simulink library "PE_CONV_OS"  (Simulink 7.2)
settings: Solver=ode45  SolverMode=SingleTasking  StartTime=0.0  StopTime=10.0  RelTol=1e-3
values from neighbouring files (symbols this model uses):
  C = 10e-3*1    (= 0.01)    [INIT_B6_2L_3Ph_IGBT_OS.m]    (also in INIT_B6_3L_3Ph_IGBT_OS.m; INIT_MMC_100L.m = 0.005; INIT_MMC_200L.m = 0.005; INIT_MMC_20L.m)
  FS = 900    [INIT_B6_2L_3Ph_IGBT_OS.m]    (also in INIT_B6_3L_3Ph_IGBT_OS.m; INIT_PWM_2L.m = 1000; INIT_PWM_3L.m = 1000; INIT_PWM_Con.m = 1000)
  LN = 2e-3    (= 0.002)    [INIT_PWM_2L.m]    (also in INIT_PWM_3L.m; INIT_PWM_Con.m; INIT_MMC_100L.m = 0.025; INIT_MMC_200L.m = 0.025)
  LS = 1e-3    (= 0.001)    [INIT_B6_2L_3Ph_IGBT_OS.m]    (also in INIT_B6_3L_3Ph_IGBT_OS.m; INIT_MMC_100L.m = 0.025; INIT_MMC_200L.m = 0.025; INIT_MMC_20L.m = 0.0025)
  LT = LN    (= 0.025)    [INIT_MMC_100L.m]    (also in INIT_MMC_200L.m; INIT_MMC_20L.m = 0.002; INIT_MMC_400L.m)
  Nc = 100    [INIT_MMC_100L.m]    (also in INIT_MMC_200L.m = 200; INIT_MMC_20L.m = 20; INIT_MMC_400L.m = 400)
  NT = sqrt(3)*340/400    [INIT_MMC_100L.m]    (also in INIT_MMC_200L.m; INIT_MMC_20L.m = sqrt(3); INIT_MMC_400L.m)
  Rg = 1e-3    (= 0.001)    [INIT_MMC_100L.m]    (also in INIT_MMC_200L.m; INIT_MMC_20L.m; INIT_MMC_400L.m)
  RN = 0.1    [INIT_PWM_2L.m]    (also in INIT_PWM_3L.m; INIT_PWM_Con.m; INIT_MMC_100L.m; INIT_MMC_200L.m)
  RT = RN    (= 0.1)    [INIT_MMC_100L.m]    (also in INIT_MMC_200L.m; INIT_MMC_20L.m; INIT_MMC_400L.m)
  UC0 = 600    [INIT_B6_2L_3Ph_IGBT_OS.m]    (also in INIT_B6_3L_3Ph_IGBT_OS.m = 500; INIT_MMC_100L.m = 6800; INIT_MMC_200L.m = 3400; INIT_MMC_20L.m = 5000)
undefined symbols (not defined in the file or in its folder): A, DT, FT, L, O1, O2, PHT, T, Td
libraries: simulink_extras x2
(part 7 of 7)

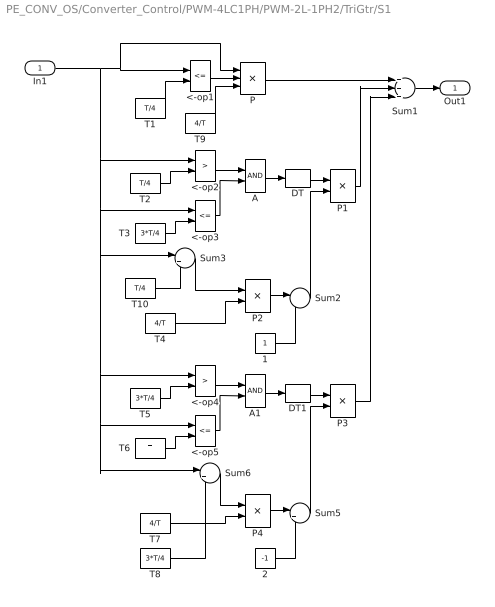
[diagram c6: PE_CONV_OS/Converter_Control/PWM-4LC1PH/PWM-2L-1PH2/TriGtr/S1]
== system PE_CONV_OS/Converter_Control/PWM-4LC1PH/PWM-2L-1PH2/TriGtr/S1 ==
  In1 : Inport  OutDataType=sfix(16)  OutScaling=2^0
  1 : Constant  OutDataType=sfix(16)  OutScaling=2^0
  2 : Constant  Value=-1  OutDataType=sfix(16)  OutScaling=2^0
  <-op1 : RelationalOperator  Operator=<=
  <-op2 : RelationalOperator  Operator=>
  <-op3 : RelationalOperator  Operator=<=
  <-op4 : RelationalOperator  Operator=>
  <-op5 : RelationalOperator  Operator=<=
  A : Logic  AllPortsSameDT=off
  A1 : Logic  AllPortsSameDT=off
  DT : DataTypeConversion
  DT1 : DataTypeConversion
  P : Product  Inputs=3  OutDataType=sfix(16)  OutScaling=2^0
  P{1..4} (4 alike) : Product  OutDataType=sfix(16)  OutScaling=2^0
  Sum1 : Sum  Inputs=+++  OutDataType=sfix(16)  OutScaling=2^0
  Sum2 : Sum  Inputs=|-+  OutDataType=sfix(16)  OutScaling=2^0
  Sum3 : Sum  Inputs=|+-  OutDataType=sfix(16)  OutScaling=2^0
  Sum5 : Sum  Inputs=|++  OutDataType=sfix(16)  OutScaling=2^0
  Sum6 : Sum  Inputs=|+-  OutDataType=sfix(16)  OutScaling=2^0
  T1 : Constant  Value=T/4  OutDataType=sfix(16)  OutScaling=2^0
  T10 : Constant  Value=T/4  OutDataType=sfix(16)  OutScaling=2^0
  T2 : Constant  Value=T/4  OutDataType=sfix(16)  OutScaling=2^0
  T3 : Constant  Value=3*T/4  OutDataType=sfix(16)  OutScaling=2^0
  T4 : Constant  Value=4/T  OutDataType=sfix(16)  OutScaling=2^0
  T5 : Constant  Value=3*T/4  OutDataType=sfix(16)  OutScaling=2^0
  T6 : Constant  Value=T  OutDataType=sfix(16)  OutScaling=2^0
  T7 : Constant  Value=4/T  OutDataType=sfix(16)  OutScaling=2^0
  T8 : Constant  Value=3*T/4  OutDataType=sfix(16)  OutScaling=2^0
  T9 : Constant  Value=4/T  OutDataType=sfix(16)  OutScaling=2^0
  Out1 : Outport
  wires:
  T10/1 -> Sum3/2
  T9/1 -> P/3
  DT1/1 -> P3/1
  DT/1 -> P1/1
  T1/1 -> <-op1/2
  <-op1/1 -> P/2
  P/1 -> Sum1/1
  T2/1 -> <-op2/2
  <-op2/1 -> A/1
  T3/1 -> <-op3/2
  <-op3/1 -> A/2
  A/1 -> DT/1
  T4/1 -> P2/2
  Sum3/1 -> P2/1
  In1/1 -> <-op2/1, <-op3/1, Sum3/1, <-op4/1, <-op5/1, Sum6/1, <-op1/1, P/1
  P1/1 -> Sum1/2
  P2/1 -> Sum2/1
  1/1 -> Sum2/2
  Sum2/1 -> P1/2
  T5/1 -> <-op4/2
  <-op4/1 -> A1/1
  T6/1 -> <-op5/2
  <-op5/1 -> A1/2
  A1/1 -> DT1/1
  T7/1 -> P4/2
  Sum6/1 -> P4/1
  P4/1 -> Sum5/1
  2/1 -> Sum5/2
  Sum5/1 -> P3/2
  T8/1 -> Sum6/2
  P3/1 -> Sum1/3
  Sum1/1 -> Out1/1

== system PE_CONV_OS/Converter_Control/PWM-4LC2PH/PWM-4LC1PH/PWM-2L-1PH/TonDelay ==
  s1 : Inport  Orientation=down  OutDataType=sfix(16)  OutScaling=2^0
  Int : Integrator  ExternalReset=falling
  Rel1 : Relay  OnSwitchValue=DT  OutDataType=sfix(16)  OutScaling=2^0
  s1d : Outport  InitialOutput=0
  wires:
  Rel1/1 -> s1d/1
  s1/1 -> Int/1, Int/2
  Int/1 -> Rel1/1

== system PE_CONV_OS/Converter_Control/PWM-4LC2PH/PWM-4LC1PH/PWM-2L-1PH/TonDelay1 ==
  s1 : Inport  Orientation=down  OutDataType=sfix(16)  OutScaling=2^0
  Int : Integrator  ExternalReset=falling
  Rel1 : Relay  OnSwitchValue=DT  OutDataType=sfix(16)  OutScaling=2^0
  s1d : Outport  InitialOutput=0
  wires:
  Rel1/1 -> s1d/1
  s1/1 -> Int/1, Int/2
  Int/1 -> Rel1/1

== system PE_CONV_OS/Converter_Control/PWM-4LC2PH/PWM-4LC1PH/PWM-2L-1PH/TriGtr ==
  Clock : Clock
  S1 : Subsystem
  Sum : Sum  OutDataType=sfix(16)  OutScaling=2^0
  T : Constant  Value=T  OutDataType=sfix(16)  OutScaling=2^0
  Td : Constant  Value=Td  OutDataType=sfix(16)  OutScaling=2^0
  mod : Math  Operator=mod
  O : Outport  InitialOutput=0
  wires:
  Td/1 -> Sum/2
  Sum/1 -> mod/1
  T/1 -> mod/2
  Clock/1 -> Sum/1
  S1/1(Out1) -> O/1
  mod/1 -> S1/1(In1)

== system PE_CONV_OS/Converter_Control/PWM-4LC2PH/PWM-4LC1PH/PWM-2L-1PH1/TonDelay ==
  s1 : Inport  Orientation=down  OutDataType=sfix(16)  OutScaling=2^0
  Int : Integrator  ExternalReset=falling
  Rel1 : Relay  OnSwitchValue=DT  OutDataType=sfix(16)  OutScaling=2^0
  s1d : Outport  InitialOutput=0
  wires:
  Int/1 -> Rel1/1
  s1/1 -> Int/2, Int/1
  Rel1/1 -> s1d/1

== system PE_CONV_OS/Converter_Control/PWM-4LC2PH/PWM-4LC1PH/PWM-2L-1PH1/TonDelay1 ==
  s1 : Inport  Orientation=down  OutDataType=sfix(16)  OutScaling=2^0
  Int : Integrator  ExternalReset=falling
  Rel1 : Relay  OnSwitchValue=DT  OutDataType=sfix(16)  OutScaling=2^0
  s1d : Outport  InitialOutput=0
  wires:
  Int/1 -> Rel1/1
  s1/1 -> Int/2, Int/1
  Rel1/1 -> s1d/1

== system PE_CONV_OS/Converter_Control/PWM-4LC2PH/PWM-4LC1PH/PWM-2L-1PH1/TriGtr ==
  Clock : Clock
  S1 : Subsystem
  Sum : Sum  OutDataType=sfix(16)  OutScaling=2^0
  T : Constant  Value=T  OutDataType=sfix(16)  OutScaling=2^0
  Td : Constant  Value=Td  OutDataType=sfix(16)  OutScaling=2^0
  mod : Math  Operator=mod
  O : Outport  InitialOutput=0
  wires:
  mod/1 -> S1/1(In1)
  S1/1(Out1) -> O/1
  Clock/1 -> Sum/1
  T/1 -> mod/2
  Sum/1 -> mod/1
  Td/1 -> Sum/2

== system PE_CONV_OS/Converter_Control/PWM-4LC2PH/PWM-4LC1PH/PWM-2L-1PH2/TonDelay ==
  s1 : Inport  Orientation=down  OutDataType=sfix(16)  OutScaling=2^0
  Int : Integrator  ExternalReset=falling
  Rel1 : Relay  OnSwitchValue=DT  OutDataType=sfix(16)  OutScaling=2^0
  s1d : Outport  InitialOutput=0
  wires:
  Rel1/1 -> s1d/1
  s1/1 -> Int/1, Int/2
  Int/1 -> Rel1/1

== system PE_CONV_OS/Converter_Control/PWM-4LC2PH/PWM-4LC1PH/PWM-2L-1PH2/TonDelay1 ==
  s1 : Inport  Orientation=down  OutDataType=sfix(16)  OutScaling=2^0
  Int : Integrator  ExternalReset=falling
  Rel1 : Relay  OnSwitchValue=DT  OutDataType=sfix(16)  OutScaling=2^0
  s1d : Outport  InitialOutput=0
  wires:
  Rel1/1 -> s1d/1
  s1/1 -> Int/1, Int/2
  Int/1 -> Rel1/1

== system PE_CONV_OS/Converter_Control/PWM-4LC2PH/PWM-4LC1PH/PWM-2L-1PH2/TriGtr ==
  Clock : Clock
  S1 : Subsystem
  Sum : Sum  OutDataType=sfix(16)  OutScaling=2^0
  T : Constant  Value=T  OutDataType=sfix(16)  OutScaling=2^0
  Td : Constant  Value=Td  OutDataType=sfix(16)  OutScaling=2^0
  mod : Math  Operator=mod
  O : Outport  InitialOutput=0
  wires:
  Td/1 -> Sum/2
  Sum/1 -> mod/1
  T/1 -> mod/2
  Clock/1 -> Sum/1
  S1/1(Out1) -> O/1
  mod/1 -> S1/1(In1)

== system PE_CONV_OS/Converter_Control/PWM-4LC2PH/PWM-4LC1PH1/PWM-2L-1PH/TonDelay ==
  s1 : Inport  Orientation=down  OutDataType=sfix(16)  OutScaling=2^0
  Int : Integrator  ExternalReset=falling
  Rel1 : Relay  OnSwitchValue=DT  OutDataType=sfix(16)  OutScaling=2^0
  s1d : Outport  InitialOutput=0
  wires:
  Int/1 -> Rel1/1
  s1/1 -> Int/2, Int/1
  Rel1/1 -> s1d/1

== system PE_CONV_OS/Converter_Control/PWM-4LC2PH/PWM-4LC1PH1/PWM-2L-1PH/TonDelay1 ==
  s1 : Inport  Orientation=down  OutDataType=sfix(16)  OutScaling=2^0
  Int : Integrator  ExternalReset=falling
  Rel1 : Relay  OnSwitchValue=DT  OutDataType=sfix(16)  OutScaling=2^0
  s1d : Outport  InitialOutput=0
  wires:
  Int/1 -> Rel1/1
  s1/1 -> Int/2, Int/1
  Rel1/1 -> s1d/1

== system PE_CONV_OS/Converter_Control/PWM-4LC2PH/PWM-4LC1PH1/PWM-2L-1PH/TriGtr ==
  Clock : Clock
  S1 : Subsystem
  Sum : Sum  OutDataType=sfix(16)  OutScaling=2^0
  T : Constant  Value=T  OutDataType=sfix(16)  OutScaling=2^0
  Td : Constant  Value=Td  OutDataType=sfix(16)  OutScaling=2^0
  mod : Math  Operator=mod
  O : Outport  InitialOutput=0
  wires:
  mod/1 -> S1/1(In1)
  S1/1(Out1) -> O/1
  Clock/1 -> Sum/1
  T/1 -> mod/2
  Sum/1 -> mod/1
  Td/1 -> Sum/2

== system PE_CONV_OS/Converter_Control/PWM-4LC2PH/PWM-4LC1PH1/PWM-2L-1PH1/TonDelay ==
  s1 : Inport  Orientation=down  OutDataType=sfix(16)  OutScaling=2^0
  Int : Integrator  ExternalReset=falling
  Rel1 : Relay  OnSwitchValue=DT  OutDataType=sfix(16)  OutScaling=2^0
  s1d : Outport  InitialOutput=0
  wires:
  Rel1/1 -> s1d/1
  s1/1 -> Int/1, Int/2
  Int/1 -> Rel1/1

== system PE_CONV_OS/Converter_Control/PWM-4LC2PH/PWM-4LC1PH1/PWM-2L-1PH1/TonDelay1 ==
  s1 : Inport  Orientation=down  OutDataType=sfix(16)  OutScaling=2^0
  Int : Integrator  ExternalReset=falling
  Rel1 : Relay  OnSwitchValue=DT  OutDataType=sfix(16)  OutScaling=2^0
  s1d : Outport  InitialOutput=0
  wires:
  Rel1/1 -> s1d/1
  s1/1 -> Int/1, Int/2
  Int/1 -> Rel1/1

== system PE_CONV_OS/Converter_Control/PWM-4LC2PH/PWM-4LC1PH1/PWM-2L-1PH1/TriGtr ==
  Clock : Clock
  S1 : Subsystem
  Sum : Sum  OutDataType=sfix(16)  OutScaling=2^0
  T : Constant  Value=T  OutDataType=sfix(16)  OutScaling=2^0
  Td : Constant  Value=Td  OutDataType=sfix(16)  OutScaling=2^0
  mod : Math  Operator=mod
  O : Outport  InitialOutput=0
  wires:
  Td/1 -> Sum/2
  Sum/1 -> mod/1
  T/1 -> mod/2
  Clock/1 -> Sum/1
  S1/1(Out1) -> O/1
  mod/1 -> S1/1(In1)

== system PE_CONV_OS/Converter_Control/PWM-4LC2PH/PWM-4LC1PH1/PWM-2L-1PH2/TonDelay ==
  s1 : Inport  Orientation=down  OutDataType=sfix(16)  OutScaling=2^0
  Int : Integrator  ExternalReset=falling
  Rel1 : Relay  OnSwitchValue=DT  OutDataType=sfix(16)  OutScaling=2^0
  s1d : Outport  InitialOutput=0
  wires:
  Int/1 -> Rel1/1
  s1/1 -> Int/2, Int/1
  Rel1/1 -> s1d/1

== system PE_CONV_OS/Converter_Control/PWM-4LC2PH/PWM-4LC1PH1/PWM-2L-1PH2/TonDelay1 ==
  s1 : Inport  Orientation=down  OutDataType=sfix(16)  OutScaling=2^0
  Int : Integrator  ExternalReset=falling
  Rel1 : Relay  OnSwitchValue=DT  OutDataType=sfix(16)  OutScaling=2^0
  s1d : Outport  InitialOutput=0
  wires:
  Int/1 -> Rel1/1
  s1/1 -> Int/2, Int/1
  Rel1/1 -> s1d/1

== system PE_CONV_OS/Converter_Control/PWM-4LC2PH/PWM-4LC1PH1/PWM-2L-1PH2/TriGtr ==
  Clock : Clock
  S1 : Subsystem
  Sum : Sum  OutDataType=sfix(16)  OutScaling=2^0
  T : Constant  Value=T  OutDataType=sfix(16)  OutScaling=2^0
  Td : Constant  Value=Td  OutDataType=sfix(16)  OutScaling=2^0
  mod : Math  Operator=mod
  O : Outport  InitialOutput=0
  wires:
  mod/1 -> S1/1(In1)
  S1/1(Out1) -> O/1
  Clock/1 -> Sum/1
  T/1 -> mod/2
  Sum/1 -> mod/1
  Td/1 -> Sum/2

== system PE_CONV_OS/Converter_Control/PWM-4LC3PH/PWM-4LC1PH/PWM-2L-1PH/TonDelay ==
  s1 : Inport  Orientation=down  OutDataType=sfix(16)  OutScaling=2^0
  Int : Integrator  ExternalReset=falling
  Rel1 : Relay  OnSwitchValue=DT  OutDataType=sfix(16)  OutScaling=2^0
  s1d : Outport  InitialOutput=0
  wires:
  Rel1/1 -> s1d/1
  s1/1 -> Int/1, Int/2
  Int/1 -> Rel1/1

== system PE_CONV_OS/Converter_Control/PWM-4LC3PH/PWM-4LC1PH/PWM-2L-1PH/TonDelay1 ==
  s1 : Inport  Orientation=down  OutDataType=sfix(16)  OutScaling=2^0
  Int : Integrator  ExternalReset=falling
  Rel1 : Relay  OnSwitchValue=DT  OutDataType=sfix(16)  OutScaling=2^0
  s1d : Outport  InitialOutput=0
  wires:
  Rel1/1 -> s1d/1
  s1/1 -> Int/1, Int/2
  Int/1 -> Rel1/1

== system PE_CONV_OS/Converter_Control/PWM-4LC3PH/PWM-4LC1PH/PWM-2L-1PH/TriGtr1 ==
  Clock : Clock
  S1 : Subsystem
  Sum : Sum  OutDataType=sfix(16)  OutScaling=2^0
  T : Constant  Value=T  OutDataType=sfix(16)  OutScaling=2^0
  Td : Constant  Value=Td  OutDataType=sfix(16)  OutScaling=2^0
  mod : Math  Operator=mod
  O : Outport  InitialOutput=0
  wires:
  Td/1 -> Sum/2
  Sum/1 -> mod/1
  T/1 -> mod/2
  Clock/1 -> Sum/1
  S1/1(O1) -> O/1
  mod/1 -> S1/1(I1)

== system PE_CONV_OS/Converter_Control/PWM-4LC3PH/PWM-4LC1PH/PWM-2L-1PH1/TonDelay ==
  s1 : Inport  Orientation=down  OutDataType=sfix(16)  OutScaling=2^0
  Int : Integrator  ExternalReset=falling
  Rel1 : Relay  OnSwitchValue=DT  OutDataType=sfix(16)  OutScaling=2^0
  s1d : Outport  InitialOutput=0
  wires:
  Int/1 -> Rel1/1
  s1/1 -> Int/2, Int/1
  Rel1/1 -> s1d/1

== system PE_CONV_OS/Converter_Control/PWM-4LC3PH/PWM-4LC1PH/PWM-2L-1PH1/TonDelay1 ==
  s1 : Inport  Orientation=down  OutDataType=sfix(16)  OutScaling=2^0
  Int : Integrator  ExternalReset=falling
  Rel1 : Relay  OnSwitchValue=DT  OutDataType=sfix(16)  OutScaling=2^0
  s1d : Outport  InitialOutput=0
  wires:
  Int/1 -> Rel1/1
  s1/1 -> Int/2, Int/1
  Rel1/1 -> s1d/1

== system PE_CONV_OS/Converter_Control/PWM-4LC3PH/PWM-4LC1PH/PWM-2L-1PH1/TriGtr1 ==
  Clock : Clock
  S1 : Subsystem
  Sum : Sum  OutDataType=sfix(16)  OutScaling=2^0
  T : Constant  Value=T  OutDataType=sfix(16)  OutScaling=2^0
  Td : Constant  Value=Td  OutDataType=sfix(16)  OutScaling=2^0
  mod : Math  Operator=mod
  O : Outport  InitialOutput=0
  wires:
  mod/1 -> S1/1(I1)
  S1/1(O1) -> O/1
  Clock/1 -> Sum/1
  T/1 -> mod/2
  Sum/1 -> mod/1
  Td/1 -> Sum/2

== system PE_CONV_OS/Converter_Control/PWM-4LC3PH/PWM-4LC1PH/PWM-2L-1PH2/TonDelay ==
  s1 : Inport  Orientation=down  OutDataType=sfix(16)  OutScaling=2^0
  Int : Integrator  ExternalReset=falling
  Rel1 : Relay  OnSwitchValue=DT  OutDataType=sfix(16)  OutScaling=2^0
  s1d : Outport  InitialOutput=0
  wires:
  Rel1/1 -> s1d/1
  s1/1 -> Int/1, Int/2
  Int/1 -> Rel1/1

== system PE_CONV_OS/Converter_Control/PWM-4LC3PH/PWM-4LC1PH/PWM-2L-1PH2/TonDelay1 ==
  s1 : Inport  Orientation=down  OutDataType=sfix(16)  OutScaling=2^0
  Int : Integrator  ExternalReset=falling
  Rel1 : Relay  OnSwitchValue=DT  OutDataType=sfix(16)  OutScaling=2^0
  s1d : Outport  InitialOutput=0
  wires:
  Rel1/1 -> s1d/1
  s1/1 -> Int/1, Int/2
  Int/1 -> Rel1/1

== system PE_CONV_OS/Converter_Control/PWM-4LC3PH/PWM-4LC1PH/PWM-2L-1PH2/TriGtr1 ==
  Clock : Clock
  S1 : Subsystem
  Sum : Sum  OutDataType=sfix(16)  OutScaling=2^0
  T : Constant  Value=T  OutDataType=sfix(16)  OutScaling=2^0
  Td : Constant  Value=Td  OutDataType=sfix(16)  OutScaling=2^0
  mod : Math  Operator=mod
  O : Outport  InitialOutput=0
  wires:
  Td/1 -> Sum/2
  Sum/1 -> mod/1
  T/1 -> mod/2
  Clock/1 -> Sum/1
  S1/1(O1) -> O/1
  mod/1 -> S1/1(I1)

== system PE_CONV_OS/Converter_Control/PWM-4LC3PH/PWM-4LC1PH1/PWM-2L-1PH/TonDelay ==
  s1 : Inport  Orientation=down  OutDataType=sfix(16)  OutScaling=2^0
  Int : Integrator  ExternalReset=falling
  Rel1 : Relay  OnSwitchValue=DT  OutDataType=sfix(16)  OutScaling=2^0
  s1d : Outport  InitialOutput=0
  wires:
  Int/1 -> Rel1/1
  s1/1 -> Int/2, Int/1
  Rel1/1 -> s1d/1

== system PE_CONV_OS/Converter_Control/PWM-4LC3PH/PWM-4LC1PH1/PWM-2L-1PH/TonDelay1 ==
  s1 : Inport  Orientation=down  OutDataType=sfix(16)  OutScaling=2^0
  Int : Integrator  ExternalReset=falling
  Rel1 : Relay  OnSwitchValue=DT  OutDataType=sfix(16)  OutScaling=2^0
  s1d : Outport  InitialOutput=0
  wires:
  Int/1 -> Rel1/1
  s1/1 -> Int/2, Int/1
  Rel1/1 -> s1d/1

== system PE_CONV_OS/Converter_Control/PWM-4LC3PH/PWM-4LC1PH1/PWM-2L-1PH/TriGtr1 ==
  Clock : Clock
  S1 : Subsystem
  Sum : Sum  OutDataType=sfix(16)  OutScaling=2^0
  T : Constant  Value=T  OutDataType=sfix(16)  OutScaling=2^0
  Td : Constant  Value=Td  OutDataType=sfix(16)  OutScaling=2^0
  mod : Math  Operator=mod
  O : Outport  InitialOutput=0
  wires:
  mod/1 -> S1/1(I1)
  S1/1(O1) -> O/1
  Clock/1 -> Sum/1
  T/1 -> mod/2
  Sum/1 -> mod/1
  Td/1 -> Sum/2

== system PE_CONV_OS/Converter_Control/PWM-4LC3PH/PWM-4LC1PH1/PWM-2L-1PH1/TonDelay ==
  s1 : Inport  Orientation=down  OutDataType=sfix(16)  OutScaling=2^0
  Int : Integrator  ExternalReset=falling
  Rel1 : Relay  OnSwitchValue=DT  OutDataType=sfix(16)  OutScaling=2^0
  s1d : Outport  InitialOutput=0
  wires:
  Rel1/1 -> s1d/1
  s1/1 -> Int/1, Int/2
  Int/1 -> Rel1/1

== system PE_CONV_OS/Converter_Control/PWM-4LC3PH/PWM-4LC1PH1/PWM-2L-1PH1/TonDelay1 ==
  s1 : Inport  Orientation=down  OutDataType=sfix(16)  OutScaling=2^0
  Int : Integrator  ExternalReset=falling
  Rel1 : Relay  OnSwitchValue=DT  OutDataType=sfix(16)  OutScaling=2^0
  s1d : Outport  InitialOutput=0
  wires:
  Rel1/1 -> s1d/1
  s1/1 -> Int/1, Int/2
  Int/1 -> Rel1/1

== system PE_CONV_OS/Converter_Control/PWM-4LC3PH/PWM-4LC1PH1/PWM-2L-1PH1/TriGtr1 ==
  Clock : Clock
  S1 : Subsystem
  Sum : Sum  OutDataType=sfix(16)  OutScaling=2^0
  T : Constant  Value=T  OutDataType=sfix(16)  OutScaling=2^0
  Td : Constant  Value=Td  OutDataType=sfix(16)  OutScaling=2^0
  mod : Math  Operator=mod
  O : Outport  InitialOutput=0
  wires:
  Td/1 -> Sum/2
  Sum/1 -> mod/1
  T/1 -> mod/2
  Clock/1 -> Sum/1
  S1/1(O1) -> O/1
  mod/1 -> S1/1(I1)

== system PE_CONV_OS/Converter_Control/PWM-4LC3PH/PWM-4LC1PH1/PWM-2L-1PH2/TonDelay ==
  s1 : Inport  Orientation=down  OutDataType=sfix(16)  OutScaling=2^0
  Int : Integrator  ExternalReset=falling
  Rel1 : Relay  OnSwitchValue=DT  OutDataType=sfix(16)  OutScaling=2^0
  s1d : Outport  InitialOutput=0
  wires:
  Int/1 -> Rel1/1
  s1/1 -> Int/2, Int/1
  Rel1/1 -> s1d/1

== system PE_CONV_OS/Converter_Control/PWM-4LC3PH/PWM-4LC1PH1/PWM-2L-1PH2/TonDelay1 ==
  s1 : Inport  Orientation=down  OutDataType=sfix(16)  OutScaling=2^0
  Int : Integrator  ExternalReset=falling
  Rel1 : Relay  OnSwitchValue=DT  OutDataType=sfix(16)  OutScaling=2^0
  s1d : Outport  InitialOutput=0
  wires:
  Int/1 -> Rel1/1
  s1/1 -> Int/2, Int/1
  Rel1/1 -> s1d/1

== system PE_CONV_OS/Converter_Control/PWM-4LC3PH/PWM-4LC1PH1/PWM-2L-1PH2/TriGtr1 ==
  Clock : Clock
  S1 : Subsystem
  Sum : Sum  OutDataType=sfix(16)  OutScaling=2^0
  T : Constant  Value=T  OutDataType=sfix(16)  OutScaling=2^0
  Td : Constant  Value=Td  OutDataType=sfix(16)  OutScaling=2^0
  mod : Math  Operator=mod
  O : Outport  InitialOutput=0
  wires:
  mod/1 -> S1/1(I1)
  S1/1(O1) -> O/1
  Clock/1 -> Sum/1
  T/1 -> mod/2
  Sum/1 -> mod/1
  Td/1 -> Sum/2

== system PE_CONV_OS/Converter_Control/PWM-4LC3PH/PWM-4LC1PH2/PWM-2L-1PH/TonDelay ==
  s1 : Inport  Orientation=down  OutDataType=sfix(16)  OutScaling=2^0
  Int : Integrator  ExternalReset=falling
  Rel1 : Relay  OnSwitchValue=DT  OutDataType=sfix(16)  OutScaling=2^0
  s1d : Outport  InitialOutput=0
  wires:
  Rel1/1 -> s1d/1
  s1/1 -> Int/1, Int/2
  Int/1 -> Rel1/1

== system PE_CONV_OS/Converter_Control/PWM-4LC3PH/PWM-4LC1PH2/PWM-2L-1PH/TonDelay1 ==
  s1 : Inport  Orientation=down  OutDataType=sfix(16)  OutScaling=2^0
  Int : Integrator  ExternalReset=falling
  Rel1 : Relay  OnSwitchValue=DT  OutDataType=sfix(16)  OutScaling=2^0
  s1d : Outport  InitialOutput=0
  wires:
  Rel1/1 -> s1d/1
  s1/1 -> Int/1, Int/2
  Int/1 -> Rel1/1

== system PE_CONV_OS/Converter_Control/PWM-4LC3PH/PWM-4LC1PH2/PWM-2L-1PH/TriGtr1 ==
  Clock : Clock
  S1 : Subsystem
  Sum : Sum  OutDataType=sfix(16)  OutScaling=2^0
  T : Constant  Value=T  OutDataType=sfix(16)  OutScaling=2^0
  Td : Constant  Value=Td  OutDataType=sfix(16)  OutScaling=2^0
  mod : Math  Operator=mod
  O : Outport  InitialOutput=0
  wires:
  Td/1 -> Sum/2
  Sum/1 -> mod/1
  T/1 -> mod/2
  Clock/1 -> Sum/1
  S1/1(O1) -> O/1
  mod/1 -> S1/1(I1)

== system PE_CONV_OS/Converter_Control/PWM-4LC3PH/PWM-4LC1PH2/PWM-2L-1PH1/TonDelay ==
  s1 : Inport  Orientation=down  OutDataType=sfix(16)  OutScaling=2^0
  Int : Integrator  ExternalReset=falling
  Rel1 : Relay  OnSwitchValue=DT  OutDataType=sfix(16)  OutScaling=2^0
  s1d : Outport  InitialOutput=0
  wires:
  Int/1 -> Rel1/1
  s1/1 -> Int/2, Int/1
  Rel1/1 -> s1d/1

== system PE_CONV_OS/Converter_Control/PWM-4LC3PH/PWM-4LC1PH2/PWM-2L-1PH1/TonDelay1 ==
  s1 : Inport  Orientation=down  OutDataType=sfix(16)  OutScaling=2^0
  Int : Integrator  ExternalReset=falling
  Rel1 : Relay  OnSwitchValue=DT  OutDataType=sfix(16)  OutScaling=2^0
  s1d : Outport  InitialOutput=0
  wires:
  Int/1 -> Rel1/1
  s1/1 -> Int/2, Int/1
  Rel1/1 -> s1d/1

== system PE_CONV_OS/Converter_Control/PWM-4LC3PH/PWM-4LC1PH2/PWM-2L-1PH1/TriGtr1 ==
  Clock : Clock
  S1 : Subsystem
  Sum : Sum  OutDataType=sfix(16)  OutScaling=2^0
  T : Constant  Value=T  OutDataType=sfix(16)  OutScaling=2^0
  Td : Constant  Value=Td  OutDataType=sfix(16)  OutScaling=2^0
  mod : Math  Operator=mod
  O : Outport  InitialOutput=0
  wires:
  mod/1 -> S1/1(I1)
  S1/1(O1) -> O/1
  Clock/1 -> Sum/1
  T/1 -> mod/2
  Sum/1 -> mod/1
  Td/1 -> Sum/2

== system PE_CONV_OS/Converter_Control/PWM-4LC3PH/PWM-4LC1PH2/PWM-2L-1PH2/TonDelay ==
  s1 : Inport  Orientation=down  OutDataType=sfix(16)  OutScaling=2^0
  Int : Integrator  ExternalReset=falling
  Rel1 : Relay  OnSwitchValue=DT  OutDataType=sfix(16)  OutScaling=2^0
  s1d : Outport  InitialOutput=0
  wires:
  Rel1/1 -> s1d/1
  s1/1 -> Int/1, Int/2
  Int/1 -> Rel1/1

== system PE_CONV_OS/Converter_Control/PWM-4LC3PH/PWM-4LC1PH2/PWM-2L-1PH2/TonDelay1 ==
  s1 : Inport  Orientation=down  OutDataType=sfix(16)  OutScaling=2^0
  Int : Integrator  ExternalReset=falling
  Rel1 : Relay  OnSwitchValue=DT  OutDataType=sfix(16)  OutScaling=2^0
  s1d : Outport  InitialOutput=0
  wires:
  Rel1/1 -> s1d/1
  s1/1 -> Int/1, Int/2
  Int/1 -> Rel1/1

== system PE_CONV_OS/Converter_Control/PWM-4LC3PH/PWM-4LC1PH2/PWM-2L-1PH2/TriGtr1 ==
  Clock : Clock
  S1 : Subsystem
  Sum : Sum  OutDataType=sfix(16)  OutScaling=2^0
  T : Constant  Value=T  OutDataType=sfix(16)  OutScaling=2^0
  Td : Constant  Value=Td  OutDataType=sfix(16)  OutScaling=2^0
  mod : Math  Operator=mod
  O : Outport  InitialOutput=0
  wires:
  Td/1 -> Sum/2
  Sum/1 -> mod/1
  T/1 -> mod/2
  Clock/1 -> Sum/1
  S1/1(O1) -> O/1
  mod/1 -> S1/1(I1)

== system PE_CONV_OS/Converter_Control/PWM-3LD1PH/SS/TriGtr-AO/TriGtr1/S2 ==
  I1 : Inport
  Fcn : Fcn  Expr="(u* (u <=T/4) * 4/T)   +  (  (u > T/4) && ( u <=3*T/4) )* ( 1 - (u-T/4) *4/T )   +  ( (u > 3*T/4)&& (u<=T)) * ( ((u -3*T/4)* 4/T )-1 )"
  O1 : Outport
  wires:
  Fcn/1 -> O1/1
  I1/1 -> Fcn/1

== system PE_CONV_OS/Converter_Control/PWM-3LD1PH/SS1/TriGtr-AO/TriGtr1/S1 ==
  I1 : Inport
  Fcn : Fcn  Expr="(u* (u <=T/4) * 4/T)   +  (  (u > T/4) && ( u <=3*T/4) )* ( 1 - (u-T/4) *4/T )   +  ( (u > 3*T/4)&& (u<=T)) * ( ((u -3*T/4)* 4/T )-1 )"
  O1 : Outport
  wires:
  I1/1 -> Fcn/1
  Fcn/1 -> O1/1

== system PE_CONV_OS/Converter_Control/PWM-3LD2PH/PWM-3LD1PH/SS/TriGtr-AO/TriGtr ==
  Clock : Clock
  Fcn : Fcn  Expr="(u* (u <=T/4) * 4/T)   +  (  (u > T/4) && ( u <=3*T/4) )* ( 1 - (u-T/4) *4/T )   +  ( (u > 3*T/4)&& (u<=T)) * ( ((u -3*T/4)* 4/T )-1 )"
  Sum : Sum
  T : Constant  Value=T
  Td : Constant  Value=Td
  mod : Math  Operator=mod
  O : Outport  InitialOutput=0
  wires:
  Td/1 -> Sum/2
  Sum/1 -> mod/1
  T/1 -> mod/2
  Clock/1 -> Sum/1
  Fcn/1 -> O/1
  mod/1 -> Fcn/1

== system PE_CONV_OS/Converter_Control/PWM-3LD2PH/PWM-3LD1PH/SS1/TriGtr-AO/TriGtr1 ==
  Clock : Clock
  Fcn : Fcn  Expr="(u* (u <=T/4) * 4/T)   +  (  (u > T/4) && ( u <=3*T/4) )* ( 1 - (u-T/4) *4/T )   +  ( (u > 3*T/4)&& (u<=T)) * ( ((u -3*T/4)* 4/T )-1 )"
  Sum : Sum
  T : Constant  Value=T
  Td : Constant  Value=Td
  mod : Math  Operator=mod
  O : Outport  InitialOutput=0
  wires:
  mod/1 -> Fcn/1
  Fcn/1 -> O/1
  Clock/1 -> Sum/1
  T/1 -> mod/2
  Sum/1 -> mod/1
  Td/1 -> Sum/2

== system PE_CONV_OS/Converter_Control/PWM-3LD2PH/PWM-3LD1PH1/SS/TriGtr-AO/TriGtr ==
  Clock : Clock
  Fcn : Fcn  Expr="(u* (u <=T/4) * 4/T)   +  (  (u > T/4) && ( u <=3*T/4) )* ( 1 - (u-T/4) *4/T )   +  ( (u > 3*T/4)&& (u<=T)) * ( ((u -3*T/4)* 4/T )-1 )"
  Sum : Sum
  T : Constant  Value=T
  Td : Constant  Value=Td
  mod : Math  Operator=mod
  O : Outport  InitialOutput=0
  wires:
  mod/1 -> Fcn/1
  Fcn/1 -> O/1
  Clock/1 -> Sum/1
  T/1 -> mod/2
  Sum/1 -> mod/1
  Td/1 -> Sum/2

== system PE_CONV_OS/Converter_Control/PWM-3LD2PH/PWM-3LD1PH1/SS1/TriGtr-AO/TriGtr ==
  Clock : Clock
  Fcn : Fcn  Expr="(u* (u <=T/4) * 4/T)   +  (  (u > T/4) && ( u <=3*T/4) )* ( 1 - (u-T/4) *4/T )   +  ( (u > 3*T/4)&& (u<=T)) * ( ((u -3*T/4)* 4/T )-1 )"
  Sum : Sum
  T : Constant  Value=T
  Td : Constant  Value=Td
  mod : Math  Operator=mod
  O : Outport  InitialOutput=0
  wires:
  mod/1 -> Fcn/1
  Fcn/1 -> O/1
  Clock/1 -> Sum/1
  T/1 -> mod/2
  Sum/1 -> mod/1
  Td/1 -> Sum/2

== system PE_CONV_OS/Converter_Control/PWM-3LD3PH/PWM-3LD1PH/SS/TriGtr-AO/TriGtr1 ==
  Clock : Clock
  S2 : Subsystem
  Sum : Sum  OutDataType=sfix(16)  OutScaling=2^0
  T : Constant  Value=T  OutDataType=sfix(16)  OutScaling=2^0
  Td : Constant  Value=Td  OutDataType=sfix(16)  OutScaling=2^0
  mod : Math  Operator=mod
  O : Outport  InitialOutput=0
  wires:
  mod/1 -> S2/1(I1)
  S2/1(O1) -> O/1
  Clock/1 -> Sum/1
  T/1 -> mod/2
  Sum/1 -> mod/1
  Td/1 -> Sum/2

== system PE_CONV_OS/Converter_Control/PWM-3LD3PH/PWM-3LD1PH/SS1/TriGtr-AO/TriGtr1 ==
  Clock : Clock
  S1 : Subsystem
  Sum : Sum
  T : Constant  Value=T
  Td : Constant  Value=Td
  mod : Math  Operator=mod
  O : Outport  InitialOutput=0
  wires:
  mod/1 -> S1/1(I1)
  S1/1(O1) -> O/1
  Clock/1 -> Sum/1
  T/1 -> mod/2
  Sum/1 -> mod/1
  Td/1 -> Sum/2

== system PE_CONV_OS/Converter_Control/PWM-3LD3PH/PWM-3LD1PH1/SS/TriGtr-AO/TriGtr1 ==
  Clock : Clock
  S2 : Subsystem
  Sum : Sum  OutDataType=sfix(16)  OutScaling=2^0
  T : Constant  Value=T  OutDataType=sfix(16)  OutScaling=2^0
  Td : Constant  Value=Td  OutDataType=sfix(16)  OutScaling=2^0
  mod : Math  Operator=mod
  O : Outport  InitialOutput=0
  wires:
  Td/1 -> Sum/2
  Sum/1 -> mod/1
  T/1 -> mod/2
  Clock/1 -> Sum/1
  S2/1(O1) -> O/1
  mod/1 -> S2/1(I1)

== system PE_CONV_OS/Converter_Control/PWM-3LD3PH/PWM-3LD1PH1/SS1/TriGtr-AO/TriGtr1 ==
  Clock : Clock
  S1 : Subsystem
  Sum : Sum
  T : Constant  Value=T
  Td : Constant  Value=Td
  mod : Math  Operator=mod
  O : Outport  InitialOutput=0
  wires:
  Td/1 -> Sum/2
  Sum/1 -> mod/1
  T/1 -> mod/2
  Clock/1 -> Sum/1
  S1/1(O1) -> O/1
  mod/1 -> S1/1(I1)

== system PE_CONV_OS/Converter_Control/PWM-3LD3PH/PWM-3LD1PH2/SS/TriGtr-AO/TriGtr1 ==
  Clock : Clock
  S2 : Subsystem
  Sum : Sum  OutDataType=sfix(16)  OutScaling=2^0
  T : Constant  Value=T  OutDataType=sfix(16)  OutScaling=2^0
  Td : Constant  Value=Td  OutDataType=sfix(16)  OutScaling=2^0
  mod : Math  Operator=mod
  O : Outport  InitialOutput=0
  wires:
  mod/1 -> S2/1(I1)
  S2/1(O1) -> O/1
  Clock/1 -> Sum/1
  T/1 -> mod/2
  Sum/1 -> mod/1
  Td/1 -> Sum/2

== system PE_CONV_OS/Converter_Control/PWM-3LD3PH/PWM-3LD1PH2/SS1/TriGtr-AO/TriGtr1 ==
  Clock : Clock
  S1 : Subsystem
  Sum : Sum
  T : Constant  Value=T
  Td : Constant  Value=Td
  mod : Math  Operator=mod
  O : Outport  InitialOutput=0
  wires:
  mod/1 -> S1/1(I1)
  S1/1(O1) -> O/1
  Clock/1 -> Sum/1
  T/1 -> mod/2
  Sum/1 -> mod/1
  Td/1 -> Sum/2

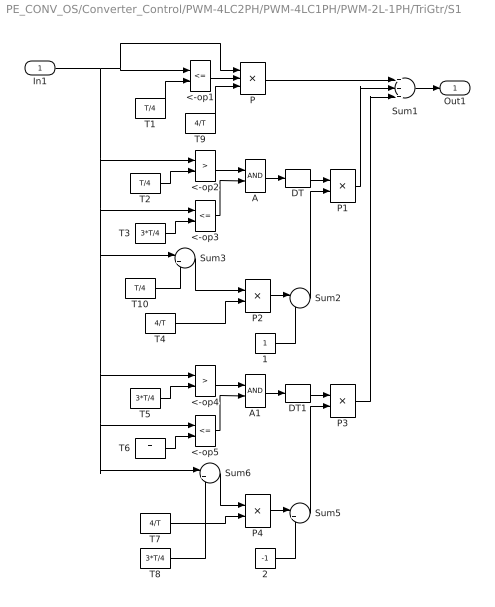
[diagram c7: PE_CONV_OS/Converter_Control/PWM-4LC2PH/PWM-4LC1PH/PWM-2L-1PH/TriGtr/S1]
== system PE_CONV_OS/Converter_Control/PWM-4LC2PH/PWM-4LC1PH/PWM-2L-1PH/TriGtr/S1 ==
  In1 : Inport  OutDataType=sfix(16)  OutScaling=2^0
  1 : Constant  OutDataType=sfix(16)  OutScaling=2^0
  2 : Constant  Value=-1  OutDataType=sfix(16)  OutScaling=2^0
  <-op1 : RelationalOperator  Operator=<=
  <-op2 : RelationalOperator  Operator=>
  <-op3 : RelationalOperator  Operator=<=
  <-op4 : RelationalOperator  Operator=>
  <-op5 : RelationalOperator  Operator=<=
  A : Logic  AllPortsSameDT=off
  A1 : Logic  AllPortsSameDT=off
  DT : DataTypeConversion
  DT1 : DataTypeConversion
  P : Product  Inputs=3  OutDataType=sfix(16)  OutScaling=2^0
  P{1..4} (4 alike) : Product  OutDataType=sfix(16)  OutScaling=2^0
  Sum1 : Sum  Inputs=+++  OutDataType=sfix(16)  OutScaling=2^0
  Sum2 : Sum  Inputs=|-+  OutDataType=sfix(16)  OutScaling=2^0
  Sum3 : Sum  Inputs=|+-  OutDataType=sfix(16)  OutScaling=2^0
  Sum5 : Sum  Inputs=|++  OutDataType=sfix(16)  OutScaling=2^0
  Sum6 : Sum  Inputs=|+-  OutDataType=sfix(16)  OutScaling=2^0
  T1 : Constant  Value=T/4  OutDataType=sfix(16)  OutScaling=2^0
  T10 : Constant  Value=T/4  OutDataType=sfix(16)  OutScaling=2^0
  T2 : Constant  Value=T/4  OutDataType=sfix(16)  OutScaling=2^0
  T3 : Constant  Value=3*T/4  OutDataType=sfix(16)  OutScaling=2^0
  T4 : Constant  Value=4/T  OutDataType=sfix(16)  OutScaling=2^0
  T5 : Constant  Value=3*T/4  OutDataType=sfix(16)  OutScaling=2^0
  T6 : Constant  Value=T  OutDataType=sfix(16)  OutScaling=2^0
  T7 : Constant  Value=4/T  OutDataType=sfix(16)  OutScaling=2^0
  T8 : Constant  Value=3*T/4  OutDataType=sfix(16)  OutScaling=2^0
  T9 : Constant  Value=4/T  OutDataType=sfix(16)  OutScaling=2^0
  Out1 : Outport
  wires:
  T10/1 -> Sum3/2
  T9/1 -> P/3
  DT1/1 -> P3/1
  DT/1 -> P1/1
  T1/1 -> <-op1/2
  <-op1/1 -> P/2
  P/1 -> Sum1/1
  T2/1 -> <-op2/2
  <-op2/1 -> A/1
  T3/1 -> <-op3/2
  <-op3/1 -> A/2
  A/1 -> DT/1
  T4/1 -> P2/2
  Sum3/1 -> P2/1
  In1/1 -> <-op2/1, <-op3/1, Sum3/1, <-op4/1, <-op5/1, Sum6/1, <-op1/1, P/1
  P1/1 -> Sum1/2
  P2/1 -> Sum2/1
  1/1 -> Sum2/2
  Sum2/1 -> P1/2
  T5/1 -> <-op4/2
  <-op4/1 -> A1/1
  T6/1 -> <-op5/2
  <-op5/1 -> A1/2
  A1/1 -> DT1/1
  T7/1 -> P4/2
  Sum6/1 -> P4/1
  P4/1 -> Sum5/1
  2/1 -> Sum5/2
  Sum5/1 -> P3/2
  T8/1 -> Sum6/2
  P3/1 -> Sum1/3
  Sum1/1 -> Out1/1

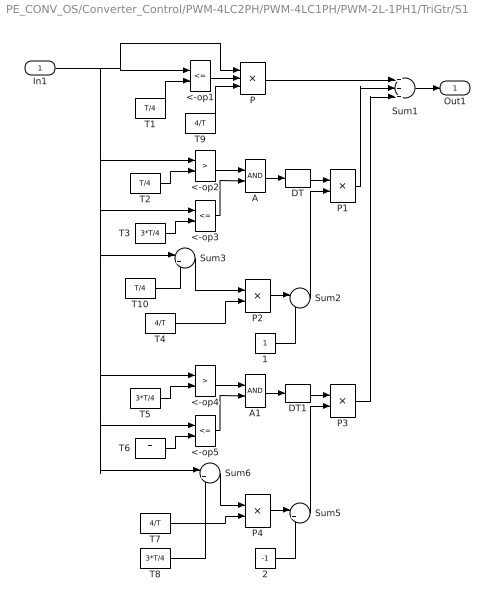
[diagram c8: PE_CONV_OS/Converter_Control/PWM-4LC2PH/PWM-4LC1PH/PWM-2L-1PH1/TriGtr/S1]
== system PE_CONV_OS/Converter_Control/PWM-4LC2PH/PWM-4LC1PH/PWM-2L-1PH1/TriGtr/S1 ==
  In1 : Inport  OutDataType=sfix(16)  OutScaling=2^0
  1 : Constant  OutDataType=sfix(16)  OutScaling=2^0
  2 : Constant  Value=-1  OutDataType=sfix(16)  OutScaling=2^0
  <-op1 : RelationalOperator  Operator=<=
  <-op2 : RelationalOperator  Operator=>
  <-op3 : RelationalOperator  Operator=<=
  <-op4 : RelationalOperator  Operator=>
  <-op5 : RelationalOperator  Operator=<=
  A : Logic  AllPortsSameDT=off
  A1 : Logic  AllPortsSameDT=off
  DT : DataTypeConversion
  DT1 : DataTypeConversion
  P : Product  Inputs=3  OutDataType=sfix(16)  OutScaling=2^0
  P{1..4} (4 alike) : Product  OutDataType=sfix(16)  OutScaling=2^0
  Sum1 : Sum  Inputs=+++  OutDataType=sfix(16)  OutScaling=2^0
  Sum2 : Sum  Inputs=|-+  OutDataType=sfix(16)  OutScaling=2^0
  Sum3 : Sum  Inputs=|+-  OutDataType=sfix(16)  OutScaling=2^0
  Sum5 : Sum  Inputs=|++  OutDataType=sfix(16)  OutScaling=2^0
  Sum6 : Sum  Inputs=|+-  OutDataType=sfix(16)  OutScaling=2^0
  T1 : Constant  Value=T/4  OutDataType=sfix(16)  OutScaling=2^0
  T10 : Constant  Value=T/4  OutDataType=sfix(16)  OutScaling=2^0
  T2 : Constant  Value=T/4  OutDataType=sfix(16)  OutScaling=2^0
  T3 : Constant  Value=3*T/4  OutDataType=sfix(16)  OutScaling=2^0
  T4 : Constant  Value=4/T  OutDataType=sfix(16)  OutScaling=2^0
  T5 : Constant  Value=3*T/4  OutDataType=sfix(16)  OutScaling=2^0
  T6 : Constant  Value=T  OutDataType=sfix(16)  OutScaling=2^0
  T7 : Constant  Value=4/T  OutDataType=sfix(16)  OutScaling=2^0
  T8 : Constant  Value=3*T/4  OutDataType=sfix(16)  OutScaling=2^0
  T9 : Constant  Value=4/T  OutDataType=sfix(16)  OutScaling=2^0
  Out1 : Outport
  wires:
  Sum1/1 -> Out1/1
  P3/1 -> Sum1/3
  T8/1 -> Sum6/2
  Sum5/1 -> P3/2
  2/1 -> Sum5/2
  P4/1 -> Sum5/1
  Sum6/1 -> P4/1
  T7/1 -> P4/2
  A1/1 -> DT1/1
  <-op5/1 -> A1/2
  T6/1 -> <-op5/2
  <-op4/1 -> A1/1
  T5/1 -> <-op4/2
  Sum2/1 -> P1/2
  1/1 -> Sum2/2
  P2/1 -> Sum2/1
  P1/1 -> Sum1/2
  In1/1 -> P/1, <-op1/1, Sum6/1, <-op5/1, <-op4/1, Sum3/1, <-op3/1, <-op2/1
  Sum3/1 -> P2/1
  T4/1 -> P2/2
  A/1 -> DT/1
  <-op3/1 -> A/2
  T3/1 -> <-op3/2
  <-op2/1 -> A/1
  T2/1 -> <-op2/2
  P/1 -> Sum1/1
  <-op1/1 -> P/2
  T1/1 -> <-op1/2
  DT/1 -> P1/1
  DT1/1 -> P3/1
  T9/1 -> P/3
  T10/1 -> Sum3/2

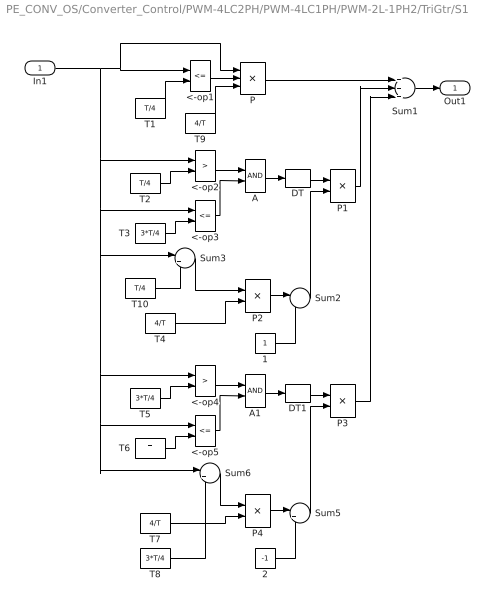
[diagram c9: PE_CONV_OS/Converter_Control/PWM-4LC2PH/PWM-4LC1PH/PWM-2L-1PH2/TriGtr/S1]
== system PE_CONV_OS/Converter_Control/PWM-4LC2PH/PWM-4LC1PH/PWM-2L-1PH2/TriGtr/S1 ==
  In1 : Inport  OutDataType=sfix(16)  OutScaling=2^0
  1 : Constant  OutDataType=sfix(16)  OutScaling=2^0
  2 : Constant  Value=-1  OutDataType=sfix(16)  OutScaling=2^0
  <-op1 : RelationalOperator  Operator=<=
  <-op2 : RelationalOperator  Operator=>
  <-op3 : RelationalOperator  Operator=<=
  <-op4 : RelationalOperator  Operator=>
  <-op5 : RelationalOperator  Operator=<=
  A : Logic  AllPortsSameDT=off
  A1 : Logic  AllPortsSameDT=off
  DT : DataTypeConversion
  DT1 : DataTypeConversion
  P : Product  Inputs=3  OutDataType=sfix(16)  OutScaling=2^0
  P{1..4} (4 alike) : Product  OutDataType=sfix(16)  OutScaling=2^0
  Sum1 : Sum  Inputs=+++  OutDataType=sfix(16)  OutScaling=2^0
  Sum2 : Sum  Inputs=|-+  OutDataType=sfix(16)  OutScaling=2^0
  Sum3 : Sum  Inputs=|+-  OutDataType=sfix(16)  OutScaling=2^0
  Sum5 : Sum  Inputs=|++  OutDataType=sfix(16)  OutScaling=2^0
  Sum6 : Sum  Inputs=|+-  OutDataType=sfix(16)  OutScaling=2^0
  T1 : Constant  Value=T/4  OutDataType=sfix(16)  OutScaling=2^0
  T10 : Constant  Value=T/4  OutDataType=sfix(16)  OutScaling=2^0
  T2 : Constant  Value=T/4  OutDataType=sfix(16)  OutScaling=2^0
  T3 : Constant  Value=3*T/4  OutDataType=sfix(16)  OutScaling=2^0
  T4 : Constant  Value=4/T  OutDataType=sfix(16)  OutScaling=2^0
  T5 : Constant  Value=3*T/4  OutDataType=sfix(16)  OutScaling=2^0
  T6 : Constant  Value=T  OutDataType=sfix(16)  OutScaling=2^0
  T7 : Constant  Value=4/T  OutDataType=sfix(16)  OutScaling=2^0
  T8 : Constant  Value=3*T/4  OutDataType=sfix(16)  OutScaling=2^0
  T9 : Constant  Value=4/T  OutDataType=sfix(16)  OutScaling=2^0
  Out1 : Outport
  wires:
  T10/1 -> Sum3/2
  T9/1 -> P/3
  DT1/1 -> P3/1
  DT/1 -> P1/1
  T1/1 -> <-op1/2
  <-op1/1 -> P/2
  P/1 -> Sum1/1
  T2/1 -> <-op2/2
  <-op2/1 -> A/1
  T3/1 -> <-op3/2
  <-op3/1 -> A/2
  A/1 -> DT/1
  T4/1 -> P2/2
  Sum3/1 -> P2/1
  In1/1 -> <-op2/1, <-op3/1, Sum3/1, <-op4/1, <-op5/1, Sum6/1, <-op1/1, P/1
  P1/1 -> Sum1/2
  P2/1 -> Sum2/1
  1/1 -> Sum2/2
  Sum2/1 -> P1/2
  T5/1 -> <-op4/2
  <-op4/1 -> A1/1
  T6/1 -> <-op5/2
  <-op5/1 -> A1/2
  A1/1 -> DT1/1
  T7/1 -> P4/2
  Sum6/1 -> P4/1
  P4/1 -> Sum5/1
  2/1 -> Sum5/2
  Sum5/1 -> P3/2
  T8/1 -> Sum6/2
  P3/1 -> Sum1/3
  Sum1/1 -> Out1/1

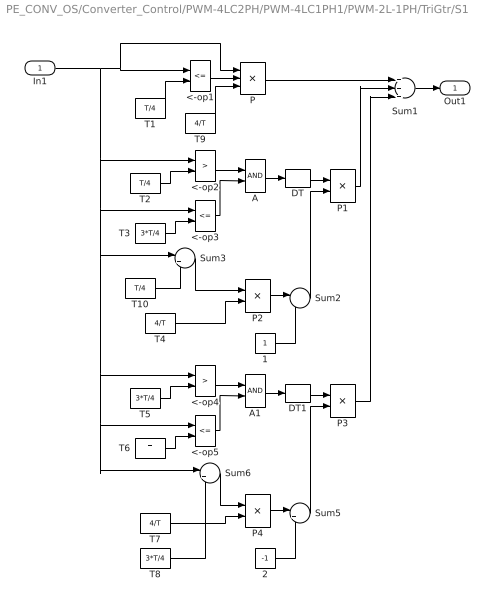
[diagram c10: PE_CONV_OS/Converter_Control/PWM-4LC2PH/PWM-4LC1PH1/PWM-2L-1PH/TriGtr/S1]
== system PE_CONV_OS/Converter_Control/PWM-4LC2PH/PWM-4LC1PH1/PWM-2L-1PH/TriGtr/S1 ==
  In1 : Inport  OutDataType=sfix(16)  OutScaling=2^0
  1 : Constant  OutDataType=sfix(16)  OutScaling=2^0
  2 : Constant  Value=-1  OutDataType=sfix(16)  OutScaling=2^0
  <-op1 : RelationalOperator  Operator=<=
  <-op2 : RelationalOperator  Operator=>
  <-op3 : RelationalOperator  Operator=<=
  <-op4 : RelationalOperator  Operator=>
  <-op5 : RelationalOperator  Operator=<=
  A : Logic  AllPortsSameDT=off
  A1 : Logic  AllPortsSameDT=off
  DT : DataTypeConversion
  DT1 : DataTypeConversion
  P : Product  Inputs=3  OutDataType=sfix(16)  OutScaling=2^0
  P{1..4} (4 alike) : Product  OutDataType=sfix(16)  OutScaling=2^0
  Sum1 : Sum  Inputs=+++  OutDataType=sfix(16)  OutScaling=2^0
  Sum2 : Sum  Inputs=|-+  OutDataType=sfix(16)  OutScaling=2^0
  Sum3 : Sum  Inputs=|+-  OutDataType=sfix(16)  OutScaling=2^0
  Sum5 : Sum  Inputs=|++  OutDataType=sfix(16)  OutScaling=2^0
  Sum6 : Sum  Inputs=|+-  OutDataType=sfix(16)  OutScaling=2^0
  T1 : Constant  Value=T/4  OutDataType=sfix(16)  OutScaling=2^0
  T10 : Constant  Value=T/4  OutDataType=sfix(16)  OutScaling=2^0
  T2 : Constant  Value=T/4  OutDataType=sfix(16)  OutScaling=2^0
  T3 : Constant  Value=3*T/4  OutDataType=sfix(16)  OutScaling=2^0
  T4 : Constant  Value=4/T  OutDataType=sfix(16)  OutScaling=2^0
  T5 : Constant  Value=3*T/4  OutDataType=sfix(16)  OutScaling=2^0
  T6 : Constant  Value=T  OutDataType=sfix(16)  OutScaling=2^0
  T7 : Constant  Value=4/T  OutDataType=sfix(16)  OutScaling=2^0
  T8 : Constant  Value=3*T/4  OutDataType=sfix(16)  OutScaling=2^0
  T9 : Constant  Value=4/T  OutDataType=sfix(16)  OutScaling=2^0
  Out1 : Outport
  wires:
  Sum1/1 -> Out1/1
  P3/1 -> Sum1/3
  T8/1 -> Sum6/2
  Sum5/1 -> P3/2
  2/1 -> Sum5/2
  P4/1 -> Sum5/1
  Sum6/1 -> P4/1
  T7/1 -> P4/2
  A1/1 -> DT1/1
  <-op5/1 -> A1/2
  T6/1 -> <-op5/2
  <-op4/1 -> A1/1
  T5/1 -> <-op4/2
  Sum2/1 -> P1/2
  1/1 -> Sum2/2
  P2/1 -> Sum2/1
  P1/1 -> Sum1/2
  In1/1 -> P/1, <-op1/1, Sum6/1, <-op5/1, <-op4/1, Sum3/1, <-op3/1, <-op2/1
  Sum3/1 -> P2/1
  T4/1 -> P2/2
  A/1 -> DT/1
  <-op3/1 -> A/2
  T3/1 -> <-op3/2
  <-op2/1 -> A/1
  T2/1 -> <-op2/2
  P/1 -> Sum1/1
  <-op1/1 -> P/2
  T1/1 -> <-op1/2
  DT/1 -> P1/1
  DT1/1 -> P3/1
  T9/1 -> P/3
  T10/1 -> Sum3/2

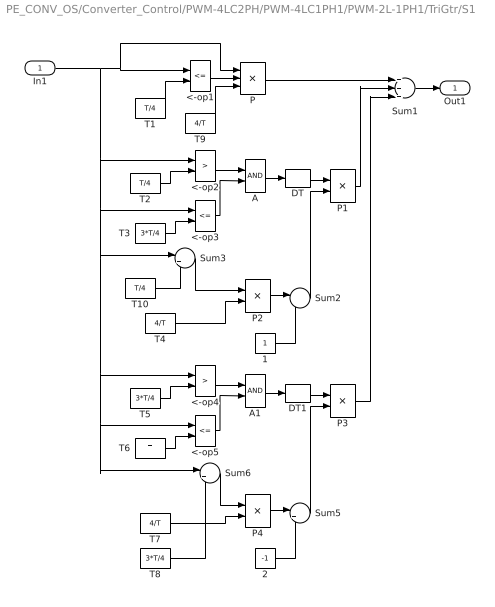
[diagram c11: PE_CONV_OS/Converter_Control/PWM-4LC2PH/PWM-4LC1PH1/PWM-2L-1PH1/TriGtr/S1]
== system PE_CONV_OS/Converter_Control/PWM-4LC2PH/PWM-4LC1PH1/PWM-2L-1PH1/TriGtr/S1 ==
  In1 : Inport  OutDataType=sfix(16)  OutScaling=2^0
  1 : Constant  OutDataType=sfix(16)  OutScaling=2^0
  2 : Constant  Value=-1  OutDataType=sfix(16)  OutScaling=2^0
  <-op1 : RelationalOperator  Operator=<=
  <-op2 : RelationalOperator  Operator=>
  <-op3 : RelationalOperator  Operator=<=
  <-op4 : RelationalOperator  Operator=>
  <-op5 : RelationalOperator  Operator=<=
  A : Logic  AllPortsSameDT=off
  A1 : Logic  AllPortsSameDT=off
  DT : DataTypeConversion
  DT1 : DataTypeConversion
  P : Product  Inputs=3  OutDataType=sfix(16)  OutScaling=2^0
  P{1..4} (4 alike) : Product  OutDataType=sfix(16)  OutScaling=2^0
  Sum1 : Sum  Inputs=+++  OutDataType=sfix(16)  OutScaling=2^0
  Sum2 : Sum  Inputs=|-+  OutDataType=sfix(16)  OutScaling=2^0
  Sum3 : Sum  Inputs=|+-  OutDataType=sfix(16)  OutScaling=2^0
  Sum5 : Sum  Inputs=|++  OutDataType=sfix(16)  OutScaling=2^0
  Sum6 : Sum  Inputs=|+-  OutDataType=sfix(16)  OutScaling=2^0
  T1 : Constant  Value=T/4  OutDataType=sfix(16)  OutScaling=2^0
  T10 : Constant  Value=T/4  OutDataType=sfix(16)  OutScaling=2^0
  T2 : Constant  Value=T/4  OutDataType=sfix(16)  OutScaling=2^0
  T3 : Constant  Value=3*T/4  OutDataType=sfix(16)  OutScaling=2^0
  T4 : Constant  Value=4/T  OutDataType=sfix(16)  OutScaling=2^0
  T5 : Constant  Value=3*T/4  OutDataType=sfix(16)  OutScaling=2^0
  T6 : Constant  Value=T  OutDataType=sfix(16)  OutScaling=2^0
  T7 : Constant  Value=4/T  OutDataType=sfix(16)  OutScaling=2^0
  T8 : Constant  Value=3*T/4  OutDataType=sfix(16)  OutScaling=2^0
  T9 : Constant  Value=4/T  OutDataType=sfix(16)  OutScaling=2^0
  Out1 : Outport
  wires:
  T10/1 -> Sum3/2
  T9/1 -> P/3
  DT1/1 -> P3/1
  DT/1 -> P1/1
  T1/1 -> <-op1/2
  <-op1/1 -> P/2
  P/1 -> Sum1/1
  T2/1 -> <-op2/2
  <-op2/1 -> A/1
  T3/1 -> <-op3/2
  <-op3/1 -> A/2
  A/1 -> DT/1
  T4/1 -> P2/2
  Sum3/1 -> P2/1
  In1/1 -> <-op2/1, <-op3/1, Sum3/1, <-op4/1, <-op5/1, Sum6/1, <-op1/1, P/1
  P1/1 -> Sum1/2
  P2/1 -> Sum2/1
  1/1 -> Sum2/2
  Sum2/1 -> P1/2
  T5/1 -> <-op4/2
  <-op4/1 -> A1/1
  T6/1 -> <-op5/2
  <-op5/1 -> A1/2
  A1/1 -> DT1/1
  T7/1 -> P4/2
  Sum6/1 -> P4/1
  P4/1 -> Sum5/1
  2/1 -> Sum5/2
  Sum5/1 -> P3/2
  T8/1 -> Sum6/2
  P3/1 -> Sum1/3
  Sum1/1 -> Out1/1

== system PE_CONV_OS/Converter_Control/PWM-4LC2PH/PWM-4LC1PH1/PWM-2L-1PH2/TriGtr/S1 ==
  In1 : Inport  OutDataType=sfix(16)  OutScaling=2^0
  1 : Constant  OutDataType=sfix(16)  OutScaling=2^0
  2 : Constant  Value=-1  OutDataType=sfix(16)  OutScaling=2^0
  <-op1 : RelationalOperator  Operator=<=
  <-op2 : RelationalOperator  Operator=>
  <-op3 : RelationalOperator  Operator=<=
  <-op4 : RelationalOperator  Operator=>
  <-op5 : RelationalOperator  Operator=<=
  A : Logic  AllPortsSameDT=off
  A1 : Logic  AllPortsSameDT=off
  DT : DataTypeConversion
  DT1 : DataTypeConversion
  P : Product  Inputs=3  OutDataType=sfix(16)  OutScaling=2^0
  P{1..4} (4 alike) : Product  OutDataType=sfix(16)  OutScaling=2^0
  Sum1 : Sum  Inputs=+++  OutDataType=sfix(16)  OutScaling=2^0
  Sum2 : Sum  Inputs=|-+  OutDataType=sfix(16)  OutScaling=2^0
  Sum3 : Sum  Inputs=|+-  OutDataType=sfix(16)  OutScaling=2^0
  Sum5 : Sum  Inputs=|++  OutDataType=sfix(16)  OutScaling=2^0
  Sum6 : Sum  Inputs=|+-  OutDataType=sfix(16)  OutScaling=2^0
  T1 : Constant  Value=T/4  OutDataType=sfix(16)  OutScaling=2^0
  T10 : Constant  Value=T/4  OutDataType=sfix(16)  OutScaling=2^0
  T2 : Constant  Value=T/4  OutDataType=sfix(16)  OutScaling=2^0
  T3 : Constant  Value=3*T/4  OutDataType=sfix(16)  OutScaling=2^0
  T4 : Constant  Value=4/T  OutDataType=sfix(16)  OutScaling=2^0
  T5 : Constant  Value=3*T/4  OutDataType=sfix(16)  OutScaling=2^0
  T6 : Constant  Value=T  OutDataType=sfix(16)  OutScaling=2^0
  T7 : Constant  Value=4/T  OutDataType=sfix(16)  OutScaling=2^0
  T8 : Constant  Value=3*T/4  OutDataType=sfix(16)  OutScaling=2^0
  T9 : Constant  Value=4/T  OutDataType=sfix(16)  OutScaling=2^0
  Out1 : Outport
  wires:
  Sum1/1 -> Out1/1
  P3/1 -> Sum1/3
  T8/1 -> Sum6/2
  Sum5/1 -> P3/2
  2/1 -> Sum5/2
  P4/1 -> Sum5/1
  Sum6/1 -> P4/1
  T7/1 -> P4/2
  A1/1 -> DT1/1
  <-op5/1 -> A1/2
  T6/1 -> <-op5/2
  <-op4/1 -> A1/1
  T5/1 -> <-op4/2
  Sum2/1 -> P1/2
  1/1 -> Sum2/2
  P2/1 -> Sum2/1
  P1/1 -> Sum1/2
  In1/1 -> P/1, <-op1/1, Sum6/1, <-op5/1, <-op4/1, Sum3/1, <-op3/1, <-op2/1
  Sum3/1 -> P2/1
  T4/1 -> P2/2
  A/1 -> DT/1
  <-op3/1 -> A/2
  T3/1 -> <-op3/2
  <-op2/1 -> A/1
  T2/1 -> <-op2/2
  P/1 -> Sum1/1
  <-op1/1 -> P/2
  T1/1 -> <-op1/2
  DT/1 -> P1/1
  DT1/1 -> P3/1
  T9/1 -> P/3
  T10/1 -> Sum3/2

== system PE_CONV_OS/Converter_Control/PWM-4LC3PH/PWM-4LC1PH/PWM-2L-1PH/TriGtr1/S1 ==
  I1 : Inport  OutDataType=sfix(16)  OutScaling=2^0
  Fcn : Fcn  Expr=u* (u <=T/4) * 4/T
  Fcn1 : Fcn  Expr="(  (u > T/4) && ( u <=3*T/4) )* ( 1 - (u-T/4) *4/T )"
  Fcn2 : Fcn  Expr=( (u > 3*T/4)&& (u<=T)) * ( ((u -3*T/4)* 4/T )-1 )
  Sum1 : Sum  Inputs=+++  OutDataType=sfix(16)  OutScaling=2^0
  O1 : Outport
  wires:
  I1/1 -> Fcn1/1, Fcn2/1, Fcn/1
  Sum1/1 -> O1/1
  Fcn/1 -> Sum1/1
  Fcn1/1 -> Sum1/2
  Fcn2/1 -> Sum1/3

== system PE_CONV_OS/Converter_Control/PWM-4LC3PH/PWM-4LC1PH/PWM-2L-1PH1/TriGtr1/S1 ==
  I1 : Inport  OutDataType=sfix(16)  OutScaling=2^0
  Fcn : Fcn  Expr=u* (u <=T/4) * 4/T
  Fcn1 : Fcn  Expr="(  (u > T/4) && ( u <=3*T/4) )* ( 1 - (u-T/4) *4/T )"
  Fcn2 : Fcn  Expr=( (u > 3*T/4)&& (u<=T)) * ( ((u -3*T/4)* 4/T )-1 )
  Sum1 : Sum  Inputs=+++  OutDataType=sfix(16)  OutScaling=2^0
  O1 : Outport
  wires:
  Fcn2/1 -> Sum1/3
  Fcn1/1 -> Sum1/2
  Fcn/1 -> Sum1/1
  Sum1/1 -> O1/1
  I1/1 -> Fcn/1, Fcn2/1, Fcn1/1

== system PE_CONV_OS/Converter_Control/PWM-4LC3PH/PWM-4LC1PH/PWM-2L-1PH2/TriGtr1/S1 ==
  I1 : Inport  OutDataType=sfix(16)  OutScaling=2^0
  Fcn : Fcn  Expr=u* (u <=T/4) * 4/T
  Fcn1 : Fcn  Expr="(  (u > T/4) && ( u <=3*T/4) )* ( 1 - (u-T/4) *4/T )"
  Fcn2 : Fcn  Expr=( (u > 3*T/4)&& (u<=T)) * ( ((u -3*T/4)* 4/T )-1 )
  Sum1 : Sum  Inputs=+++  OutDataType=sfix(16)  OutScaling=2^0
  O1 : Outport
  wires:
  I1/1 -> Fcn1/1, Fcn2/1, Fcn/1
  Sum1/1 -> O1/1
  Fcn/1 -> Sum1/1
  Fcn1/1 -> Sum1/2
  Fcn2/1 -> Sum1/3

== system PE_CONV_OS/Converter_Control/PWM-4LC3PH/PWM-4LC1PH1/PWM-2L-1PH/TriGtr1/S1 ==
  I1 : Inport  OutDataType=sfix(16)  OutScaling=2^0
  Fcn : Fcn  Expr=u* (u <=T/4) * 4/T
  Fcn1 : Fcn  Expr="(  (u > T/4) && ( u <=3*T/4) )* ( 1 - (u-T/4) *4/T )"
  Fcn2 : Fcn  Expr=( (u > 3*T/4)&& (u<=T)) * ( ((u -3*T/4)* 4/T )-1 )
  Sum1 : Sum  Inputs=+++  OutDataType=sfix(16)  OutScaling=2^0
  O1 : Outport
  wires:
  Fcn2/1 -> Sum1/3
  Fcn1/1 -> Sum1/2
  Fcn/1 -> Sum1/1
  Sum1/1 -> O1/1
  I1/1 -> Fcn/1, Fcn2/1, Fcn1/1

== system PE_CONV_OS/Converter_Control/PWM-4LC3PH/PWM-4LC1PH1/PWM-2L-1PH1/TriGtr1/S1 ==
  I1 : Inport  OutDataType=sfix(16)  OutScaling=2^0
  Fcn : Fcn  Expr=u* (u <=T/4) * 4/T
  Fcn1 : Fcn  Expr="(  (u > T/4) && ( u <=3*T/4) )* ( 1 - (u-T/4) *4/T )"
  Fcn2 : Fcn  Expr=( (u > 3*T/4)&& (u<=T)) * ( ((u -3*T/4)* 4/T )-1 )
  Sum1 : Sum  Inputs=+++  OutDataType=sfix(16)  OutScaling=2^0
  O1 : Outport
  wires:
  I1/1 -> Fcn1/1, Fcn2/1, Fcn/1
  Sum1/1 -> O1/1
  Fcn/1 -> Sum1/1
  Fcn1/1 -> Sum1/2
  Fcn2/1 -> Sum1/3

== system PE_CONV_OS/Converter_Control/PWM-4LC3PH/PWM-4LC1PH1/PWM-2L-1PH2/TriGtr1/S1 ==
  I1 : Inport  OutDataType=sfix(16)  OutScaling=2^0
  Fcn : Fcn  Expr=u* (u <=T/4) * 4/T
  Fcn1 : Fcn  Expr="(  (u > T/4) && ( u <=3*T/4) )* ( 1 - (u-T/4) *4/T )"
  Fcn2 : Fcn  Expr=( (u > 3*T/4)&& (u<=T)) * ( ((u -3*T/4)* 4/T )-1 )
  Sum1 : Sum  Inputs=+++  OutDataType=sfix(16)  OutScaling=2^0
  O1 : Outport
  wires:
  Fcn2/1 -> Sum1/3
  Fcn1/1 -> Sum1/2
  Fcn/1 -> Sum1/1
  Sum1/1 -> O1/1
  I1/1 -> Fcn/1, Fcn2/1, Fcn1/1

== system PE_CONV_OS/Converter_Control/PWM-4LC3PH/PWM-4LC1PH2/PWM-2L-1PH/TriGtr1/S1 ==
  I1 : Inport  OutDataType=sfix(16)  OutScaling=2^0
  Fcn : Fcn  Expr=u* (u <=T/4) * 4/T
  Fcn1 : Fcn  Expr="(  (u > T/4) && ( u <=3*T/4) )* ( 1 - (u-T/4) *4/T )"
  Fcn2 : Fcn  Expr=( (u > 3*T/4)&& (u<=T)) * ( ((u -3*T/4)* 4/T )-1 )
  Sum1 : Sum  Inputs=+++  OutDataType=sfix(16)  OutScaling=2^0
  O1 : Outport
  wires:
  I1/1 -> Fcn1/1, Fcn2/1, Fcn/1
  Sum1/1 -> O1/1
  Fcn/1 -> Sum1/1
  Fcn1/1 -> Sum1/2
  Fcn2/1 -> Sum1/3

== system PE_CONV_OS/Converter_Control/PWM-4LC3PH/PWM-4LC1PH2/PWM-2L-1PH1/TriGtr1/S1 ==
  I1 : Inport  OutDataType=sfix(16)  OutScaling=2^0
  Fcn : Fcn  Expr=u* (u <=T/4) * 4/T
  Fcn1 : Fcn  Expr="(  (u > T/4) && ( u <=3*T/4) )* ( 1 - (u-T/4) *4/T )"
  Fcn2 : Fcn  Expr=( (u > 3*T/4)&& (u<=T)) * ( ((u -3*T/4)* 4/T )-1 )
  Sum1 : Sum  Inputs=+++  OutDataType=sfix(16)  OutScaling=2^0
  O1 : Outport
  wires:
  Fcn2/1 -> Sum1/3
  Fcn1/1 -> Sum1/2
  Fcn/1 -> Sum1/1
  Sum1/1 -> O1/1
  I1/1 -> Fcn/1, Fcn2/1, Fcn1/1

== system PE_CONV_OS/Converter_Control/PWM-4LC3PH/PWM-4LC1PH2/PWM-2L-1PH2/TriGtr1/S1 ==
  I1 : Inport  OutDataType=sfix(16)  OutScaling=2^0
  Fcn : Fcn  Expr=u* (u <=T/4) * 4/T
  Fcn1 : Fcn  Expr="(  (u > T/4) && ( u <=3*T/4) )* ( 1 - (u-T/4) *4/T )"
  Fcn2 : Fcn  Expr=( (u > 3*T/4)&& (u<=T)) * ( ((u -3*T/4)* 4/T )-1 )
  Sum1 : Sum  Inputs=+++  OutDataType=sfix(16)  OutScaling=2^0
  O1 : Outport
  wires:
  I1/1 -> Fcn1/1, Fcn2/1, Fcn/1
  Sum1/1 -> O1/1
  Fcn/1 -> Sum1/1
  Fcn1/1 -> Sum1/2
  Fcn2/1 -> Sum1/3

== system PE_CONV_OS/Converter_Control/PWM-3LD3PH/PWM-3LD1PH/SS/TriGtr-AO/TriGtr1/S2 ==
  I1 : Inport
  Fcn : Fcn  Expr="(u* (u <=T/4) * 4/T)   +  (  (u > T/4) && ( u <=3*T/4) )* ( 1 - (u-T/4) *4/T )   +  ( (u > 3*T/4)&& (u<=T)) * ( ((u -3*T/4)* 4/T )-1 )"
  O1 : Outport
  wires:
  I1/1 -> Fcn/1
  Fcn/1 -> O1/1

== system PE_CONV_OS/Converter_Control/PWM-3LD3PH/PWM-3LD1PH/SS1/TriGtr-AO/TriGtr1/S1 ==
  I1 : Inport
  Fcn : Fcn  Expr="(u* (u <=T/4) * 4/T)   +  (  (u > T/4) && ( u <=3*T/4) )* ( 1 - (u-T/4) *4/T )   +  ( (u > 3*T/4)&& (u<=T)) * ( ((u -3*T/4)* 4/T )-1 )"
  O1 : Outport
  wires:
  Fcn/1 -> O1/1
  I1/1 -> Fcn/1

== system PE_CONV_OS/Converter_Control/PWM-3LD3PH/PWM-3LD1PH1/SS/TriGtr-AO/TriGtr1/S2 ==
  I1 : Inport
  Fcn : Fcn  Expr="(u* (u <=T/4) * 4/T)   +  (  (u > T/4) && ( u <=3*T/4) )* ( 1 - (u-T/4) *4/T )   +  ( (u > 3*T/4)&& (u<=T)) * ( ((u -3*T/4)* 4/T )-1 )"
  O1 : Outport
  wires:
  Fcn/1 -> O1/1
  I1/1 -> Fcn/1

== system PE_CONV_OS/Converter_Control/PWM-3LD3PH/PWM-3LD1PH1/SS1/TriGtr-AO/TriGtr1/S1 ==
  I1 : Inport
  Fcn : Fcn  Expr="(u* (u <=T/4) * 4/T)   +  (  (u > T/4) && ( u <=3*T/4) )* ( 1 - (u-T/4) *4/T )   +  ( (u > 3*T/4)&& (u<=T)) * ( ((u -3*T/4)* 4/T )-1 )"
  O1 : Outport
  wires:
  I1/1 -> Fcn/1
  Fcn/1 -> O1/1

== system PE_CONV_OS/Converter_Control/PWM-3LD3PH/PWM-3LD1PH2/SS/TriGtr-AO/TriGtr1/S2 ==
  I1 : Inport
  Fcn : Fcn  Expr="(u* (u <=T/4) * 4/T)   +  (  (u > T/4) && ( u <=3*T/4) )* ( 1 - (u-T/4) *4/T )   +  ( (u > 3*T/4)&& (u<=T)) * ( ((u -3*T/4)* 4/T )-1 )"
  O1 : Outport
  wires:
  I1/1 -> Fcn/1
  Fcn/1 -> O1/1

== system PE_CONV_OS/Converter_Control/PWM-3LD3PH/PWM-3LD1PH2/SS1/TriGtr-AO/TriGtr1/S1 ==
  I1 : Inport
  Fcn : Fcn  Expr="(u* (u <=T/4) * 4/T)   +  (  (u > T/4) && ( u <=3*T/4) )* ( 1 - (u-T/4) *4/T )   +  ( (u > 3*T/4)&& (u<=T)) * ( ((u -3*T/4)* 4/T )-1 )"
  O1 : Outport
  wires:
  Fcn/1 -> O1/1
  I1/1 -> Fcn/1
